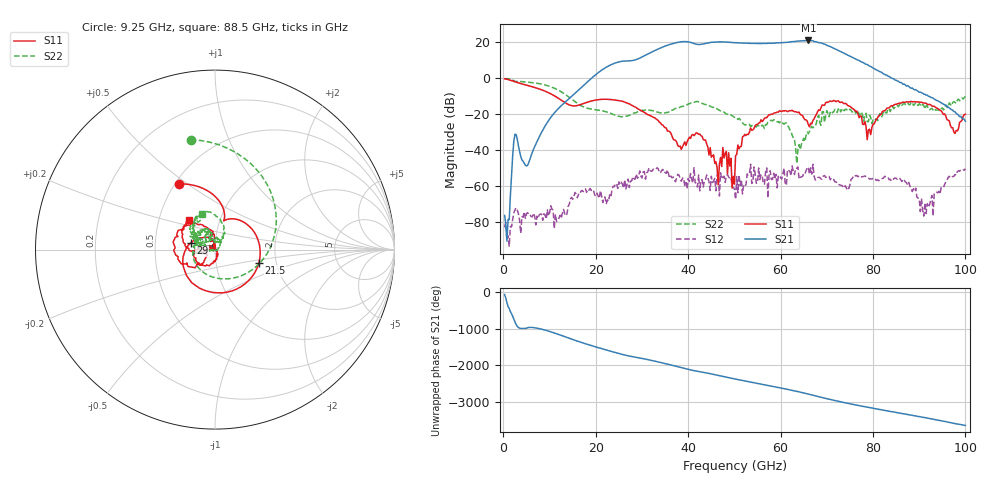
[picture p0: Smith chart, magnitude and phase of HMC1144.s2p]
! Analog Devices, Inc.
! Device:	HMC1144
! Description:	40 GHz to 70 GHz, GaAs, pHEMT, MMIC, Medium Power Amplifier
! Conditions:	Vdd = 4.0 V
!		Vgg1 = -0.49 V
!		Idd = 321.96 mA quiescent
!		Pin = -25 dBm
!		Temp = +25 C (baseplate temperature)
! Product validation unit (data sheet unit, SN 2) mounted on plate as shown on data sheet's Assembly Diagram, probed on RF probe launchers wirebonded to die pads
! Freq(GHz)	S11a(dB)	S11p(deg)	S21a(dB)	S21p(deg)	S12a(dB)	S12p(deg)	S22a(dB)	S22p(deg)
# GHz S DB R 50
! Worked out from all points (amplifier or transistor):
!   400 points, 250 MHz to 100 GHz, reference 50 ohm
!   highest |S21| = 20.8 dB at 66 GHz (marker M1)
!   |S21| within 3 dB of that: 35.15 GHz to 70.31 GHz (35.17 GHz wide, 66.7 % of centre)
!   unconditionally stable (mu >= 1): start of sweep to end of sweep
!   at 16.75 GHz: K = 1267.79, MAG = -5.3 dB, |S12| = -63.1 dB
!   at 50.25 GHz: K = 123.21, MAG = 19.6 dB, |S12| = -67.5 dB
!   at 100 GHz: K = 2387.06, MAG = -23.6 dB, |S12| = -50.5 dB
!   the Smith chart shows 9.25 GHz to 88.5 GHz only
!   S11 on the Smith chart (normalised r, x): 9.25 GHz: 0.53, +0.47; 21.5 GHz: 1.62, -0.26; 29 GHz: 0.76, +0.06; 88.5 GHz: 0.71, +0.24
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0.25  -0.47 -12.0  -76.44 -75.8  -83.09 179.1  -0.41 -12.7
9.25  -7.61 118.5  -25.72 30.4  -78.39 129.7  -4.06 102.5
17  -14.55 65.4  -4.97 57.5  -62.47 104.1  -15.69 -80.5
21.5  -11.86 -16.9  4.74 -114.2  -69.27 52.7  -18.33 -179.3
29  -17.02 165.3  10.46 12.3  -55.75 72.1  -18.86 161.9
33.5  -23.67 107.6  16.08 -106.3  -50.46 -21.1  -19.12 137.0
36.5  -32.44 89.1  19.01 164.0  -55.51 -79.7  -17.90 146.5
38.75  -38.30 134.3  20.16 93.0  -55.74 -65.3  -15.82 136.9
42.25  -31.33 120.1  18.60 -5.4  -53.98 -66.3  -13.38 100.8
46  -46.65 120.6  19.97 -100.6  -62.74 -66.1  -16.87 70.3
50.25  -43.19 3.1  19.61 147.3  -67.50 -40.2  -22.15 53.7
55.75  -23.22 -93.0  19.18 11.4  -53.70 -63.0  -27.08 89.1
60  -18.46 -136.6  19.60 -93.3  -55.47 -115.2  -24.05 74.3
63.5  -18.95 -176.1  20.44 174.8  -50.17 -72.5  -47.50 -20.9
66  -25.94 -179.4  20.83 101.2  -49.54 -134.0  -31.07 173.0
66.75  -25.56 -143.2  20.74 77.8  -53.38 -124.4  -26.92 -172.0
68.75  -16.53 -137.5  19.53 14.0  -56.17 -134.7  -26.35 -150.0
71.25  -12.96 175.6  16.82 -61.8  -56.32 -168.5  -19.34 156.7
74.75  -15.59 123.7  12.42 -156.4  -61.41 -132.1  -17.82 128.9
83.5  -16.60 177.1  0.79 -4.7  -56.59 143.3  -17.30 138.4
88.5  -13.25 131.6  -5.58 -118.4  -63.12 79.8  -13.60 110.3
100  -20.11 -173.6  -24.08 -32.1  -50.45 173.6  -10.20 118.4
